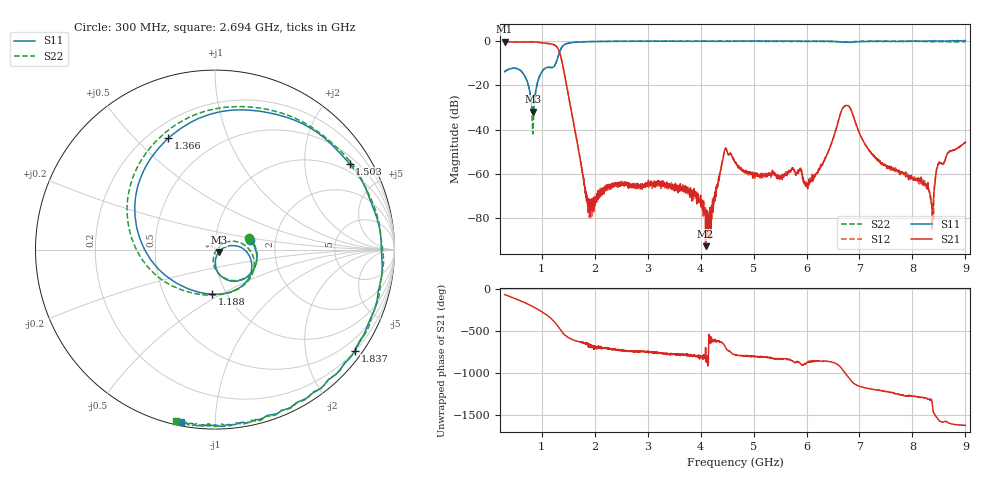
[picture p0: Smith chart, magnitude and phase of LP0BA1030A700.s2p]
!Agilent Technologies,E8358A,US41080443,A.07.50.56
!Agilent E8358A: A.07.50.56
!Date: Wednesday, March 04, 2015 10:24:19
!Correction: S11(Full 2 Port(1,2))
!S21(Full 2 Port(1,2))
!S12(Full 2 Port(1,2))
!S22(Full 2 Port(1,2))
!S2P File: Measurements: S11, S21, S12, S22:Log Frequency Sweep
# Hz S  dB  R 50
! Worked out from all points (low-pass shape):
!   3201 points, 300 MHz to 9 GHz, reference 50 ohm
!   highest |S21| = -0.33 dB at 300 MHz (marker M1); lowest = -92.7 dB at 4.094 GHz (marker M2)
!   |S21| within 3 dB of the highest: start of sweep to 1.305 GHz
!   lowest |S11| = -32.0 dB at 833.1 MHz (marker M3), VSWR 1.05, Z = 52.1 - j1.5 ohm
!   |S11| at or under -10 dB: start of sweep to 1.269 GHz
!   |S22| runs from -42.0 to 0.0 dB; largest |S21 - S12| = 0.0063
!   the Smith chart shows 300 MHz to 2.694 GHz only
!   S11 on the Smith chart (normalised r, x): 300 MHz: 1.47, +0.17; 1.188 GHz: 0.86, -0.45; 1.366 GHz: 0.28, +0.63; 1.503 GHz: 0.72, +3.28; 1.837 GHz: 0.21, -3.08; 2.694 GHz: 0.02, -0.82
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3e8  -13.90 16.2  -0.33 -71.0  -0.38 -71.1  -13.87 19.0
6.866066e8  -16.07 -75.5  -0.44 -168.9  -0.48 -168.9  -16.05 -74.8
8.331424e8  -31.96 -34.7  -0.44 146.1  -0.49 146.0  -41.90 -27.0
9.404629e8  -17.21 6.4  -0.63 108.9  -0.67 108.8  -17.35 18.1
1.064998e9  -12.32 -35.5  -0.99 59.8  -1.03 59.8  -12.31 -27.0
1.188212e9  -12.09 -93.4  -1.39 -0.8  -1.43 -0.9  -11.96 -83.7
1.285441e9  -8.87 -170.4  -2.63 -68.7  -2.67 -68.7  -8.78 -158.4
1.365725e9  -3.45 112.7  -7.60 -140.1  -7.64 -140.2  -3.46 122.7
1.502822e9  -1.02 32.6  -24.26 139.4  -24.33 139.4  -1.03 38.5
1.75137e9  -0.47 -25.3  -57.21 82.3  -57.06 83.8  -0.45 -22.5
1.837172e9  -0.35 -35.8  -68.84 70.0  -69.53 61.3  -0.35 -34.3
2.693556e9  -0.18 -101.3  -65.05 -23.9  -64.77 -28.0  -0.19 -102.8
3.203074e9  -0.10 -123.8  -63.58 -42.5  -64.40 -39.1  -0.07 -123.4
4.09446e9  -0.15 -152.8  -92.67 21.5  -75.29 -67.0  -0.05 -147.7
4.195787e9  -0.13 -154.6  -79.11 78.9  -83.68 -175.4  -0.17 -150.2
4.462582e9  -0.20 -161.4  -48.82 33.8  -48.91 31.0  -0.18 -155.9
4.651453e9  -0.19 -165.6  -54.62 -62.7  -54.65 -63.0  -0.06 -159.6
6.106022e9  -0.08 164.1  -62.28 -144.1  -61.53 -142.6  -0.25 176.3
6.747592e9  -0.56 153.1  -29.17 63.9  -29.19 64.7  -0.51 165.1
7.552286e9  -0.12 139.5  -57.53 -147.5  -57.45 -146.2  -0.22 148.3
8.292763e9  0.05 124.6  -64.02 132.4  -66.84 147.2  -0.43 129.0
9e9  0.08 111.1  -45.78 177.7  -45.65 179.2  -0.32 114.8
